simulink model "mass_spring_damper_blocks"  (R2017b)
settings: Solver=FixedStepAuto  StartTime=0.0  StopTime=10.0  FixedStep=0.01  MaxStep=0.01  RelTol=1e-3

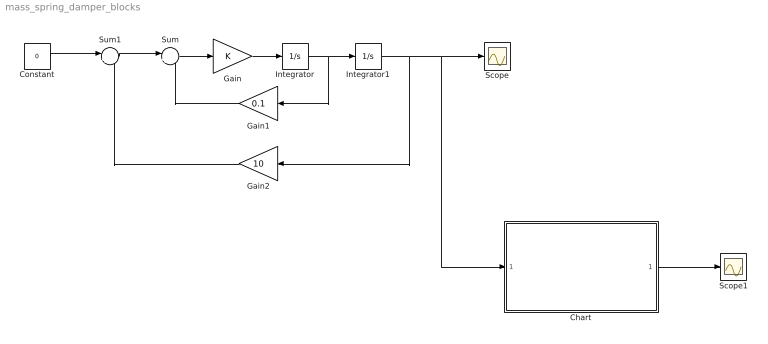
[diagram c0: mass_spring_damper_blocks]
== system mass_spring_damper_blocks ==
  Chart : Stateflow chart  TreatAsAtomicUnit=on
  Constant : Constant  Value=0
  Gain : Gain
  Gain1 : Gain  Gain=0.1
  Gain2 : Gain  Gain=10
  Integrator : Integrator
  Integrator1 : Integrator  InitialCondition=0.10
  Scope : Scope
  Scope1 : Scope
  Sum : Sum  Inputs=|+-
  Sum1 : Sum  Inputs=|+-
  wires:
  Integrator/1 -> Gain1/1, Integrator1/1
  Gain/1 -> Integrator/1
  Integrator1/1 -> Chart/1(x), Scope/1, Gain2/1
  Sum/1 -> Gain/1
  Sum1/1 -> Sum/1
  Constant/1 -> Sum1/1
  Gain1/1 -> Sum/2
  Gain2/1 -> Sum1/2
  Chart/1(y) -> Scope1/1

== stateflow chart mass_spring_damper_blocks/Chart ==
  state stateA
  state stateB
  stateB -> stateA : [x<-0.05]{y=-5}
  (default) -> stateA
  stateA -> stateB : [x>0.05]{y=5}
  data: x input; y output
